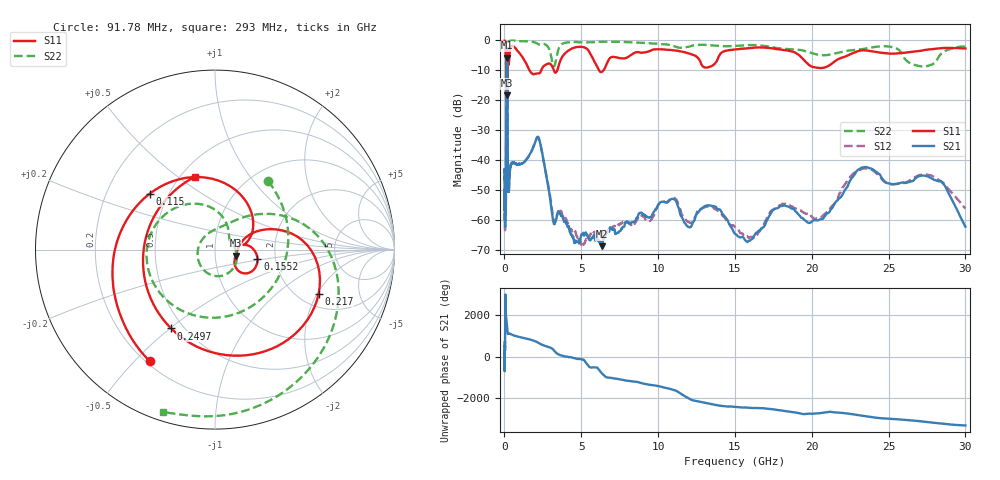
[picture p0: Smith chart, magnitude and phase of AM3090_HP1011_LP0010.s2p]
! Date/Time: Thu, Feb 28, 2019 2:05 PM
! Network Analyzer: Agilent Technologies E8364B Rev: A.07.50.67
! Sweep from 0.010 to 30.000 GHz, 1601 Points, Sweep Type: LOG
! Power Supply: 5.023 V, 0.002 A
# Hz S DB R 50
!freq MagS11 AngS11 MagS21 AngS21 MagS12 AngS12 MagS22 AngS22
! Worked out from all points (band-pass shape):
!   1601 points, 10 MHz to 30 GHz, reference 50 ohm
!   highest |S21| = -5.92 dB at 154.4 MHz (marker M1); lowest = -68.8 dB at 6.328 GHz (marker M2)
!   |S21| within 3 dB of the highest: 129.3 MHz to 187.8 MHz (58.5 MHz wide, 36.9 % of centre)
!   lowest |S11| = -18.5 dB at 185.8 MHz (marker M3), VSWR 1.27, Z = 62.7 - j4.28 ohm
!   |S11| at or under -10 dB: 1.618 GHz to 2.399 GHz (781 MHz wide, 38.9 % of centre); 3.205 GHz to 3.446 GHz (240.8 MHz wide, 7.24 % of centre); 6.144 GHz to 6.465 GHz (320.7 MHz wide, 5.09 % of centre)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
!   |S22| runs from -20.9 to -0.2 dB; largest |S21 - S12| = 0.012
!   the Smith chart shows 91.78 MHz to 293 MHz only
!   S11 on the Smith chart (normalised r, x): 91.78 MHz: 0.21, -0.55; 115 MHz: 0.39, +0.32; 155.2 MHz: 1.61, -0.17; 217 MHz: 2.54, -2.06; 249.7 MHz: 0.43, -0.50; 293 MHz: 0.59, +0.58
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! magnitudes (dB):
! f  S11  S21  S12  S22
! 10 MHz  -0.3  -43.3  -46.8  -0.6
! 38.04 MHz  -0.4  -60.8  -62.7  -1.3
! 52.66 MHz  -0.8  -50.5  -49.0  -1.4
! 91.78 MHz  -2.8  -57.5  -53.7  -6.3
! 115 MHz  -6.4  -22.8  -22.9  -8.2
! 144.7 MHz  -14.5  -6.1  -6.1  -19.4
! 154.4 MHz  -12.4  -5.9  -5.9  -16.9
! 155.2 MHz  -12.3  -5.9  -5.9  -16.7
! 185.8 MHz  -18.5  -8.4  -8.4  -19.0
! 217 MHz  -4.0  -44.3  -44.1  -2.6
! 249.7 MHz  -6.0  -50.2  -49.8  -0.8
! 293 MHz  -7.5  -49.3  -50.0  -0.5
! 550.5 MHz  -2.1  -41.1  -40.9  -0.3
! 2.084 GHz  -11.2  -32.9  -32.9  -1.0
! 3.236 GHz  -10.4  -61.4  -60.5  -8.8
! 6.328 GHz  -10.7  -68.8  -65.0  -0.6
! 7.926 GHz  -6.0  -60.7  -60.8  -0.7
! 10.76 GHz  -3.3  -53.5  -53.3  -1.7
! 15.81 GHz  -2.8  -67.5  -65.5  -1.7
! 20.51 GHz  -9.3  -59.9  -59.2  -5.0
! 23.59 GHz  -3.5  -42.4  -42.8  -2.8
! 30 GHz  -2.8  -62.3  -56.2  -2.2
